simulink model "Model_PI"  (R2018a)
settings: Solver=ode15s  StartTime=0.0  StopTime=tsim  MaxStep=0.1  RelTol=1e-5
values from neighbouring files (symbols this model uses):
  C = Fc*cpc/(Fh*cph)    [calcblock.m]    (also in calcblock2.m; calcblock3.m; eNTU.m = m.c*cp.c/(m.h*cp.h); Main.m = [zeros(1,2*N-1),1])
  d0 = [Fh, Tcin, Thin]    [Main.m]    (also in Main_OL.m; runTestCalcBlk.m; runTransf.m = [Fh; Tcin; U0; Ffeed0; m0; Tfeed0]; runTransfOL.m)
  d_step = [Fh, Tcin+0, Thin*1]    [Main_OL.m]    (also in runTestCalcBlk.m = [Fh, Tcin, Thin]; Main.m = [Fh, Tcin, Thin])
  d_tstep = 300    [Main.m]    (also in Main_OL.m = 3000; runTestCalcBlk.m; runTransf.m = [500; 50000; 70000; 130000; 50000; 50000]; runTransfOL.m = [500 5000 7000 13000])
  Fc0 = 5    [Main.m]    (also in Main_OL.m; runTestCalcBlk.m; runTransf.m; runTransfOL.m)
  Kc = 1/k*tau/(tauC+theta)    (= -0.124875124875)    [Main.m]    (also in runTransf.m = 1/kM(i)*tau(i)/(tauCM(i)+theta(i)); runTransfOL.m = 1/kM(i)*tau(i)/(tauCM(i)+theta(i)))
  nd = size(d0,2)    [Main.m]    (also in Main_OL.m; runTestCalcBlk.m; runTransf.m = size(d0,1); runTransfOL.m)
  np = size(p,2)    [Main.m]    (also in Main_OL.m; runTestCalcBlk.m; runH2Psim.m = length(param); runTransf.m)
  nu = 1    [Main.m]    (also in Main_OL.m; runTestCalcBlk.m; runH2Psim.m = length(u0); runTransf.m)
  nx = size(x0,1)    [Main.m]    (also in Main_OL.m; runTestCalcBlk.m; H2P_Turbine_driven.m = param(end); runTD.m = length(x0))
  p = [N, Fc0, rhoc, rhoh,U,A,cpc,cph]    [Main.m]    (also in Main_OL.m; runTestCalcBlk.m; NonlinearMap.m = [U;A;Fc(i);Fh;cpc;cph;Tcin;Thin]; runTransf.m = [N, Fc0, rhoc, rhoh, U0, A,cpc,cph])
  tauI = min(tau,4*(tauC+theta))    [Main.m]    (also in runTransf.m = min(tau(i), 4*(tauCM(i)+theta(i))); runTransfOL.m = min(tau(i), 4*(tauCM(i)+theta(i))))
  Thsp = Thsp0+dThsp    [Main.m]    (also in Main_OL.m = sp(j); runTestCalcBlk.m; runTransf.m = Thsp0; runTransfOL.m = Thsp0)
  Thsp0 = Thend(end)    [Main.m]    (also in Main_OL.m; runTestCalcBlk.m; runTransf.m = x0(end-1);  2.971202611676064e+02; runTransfOL.m = x0(end);  2.971202611676064e+02)
  tstep = 100    [Main.m]    (also in Main_OL.m = 500; runTransf.m = 10000; runTransfOL.m)
  x0 = [Tcend(1:N)'; Thend(1:N)']    [Main.m]    (also in Main_OL.m; runTestCalcBlk.m; runTD.m = [TE0;TD0;TSh0;MD0; MSh0;w0;TA0;0;0;0;0;0;0;0;0;0]; runBD.m = [TE0;TD0;TSh0;MD0; MSh0;w0;TA0;0;0;0;0;0;0;0;0;0])
undefined symbols (not defined in the file or in its folder): HEXode

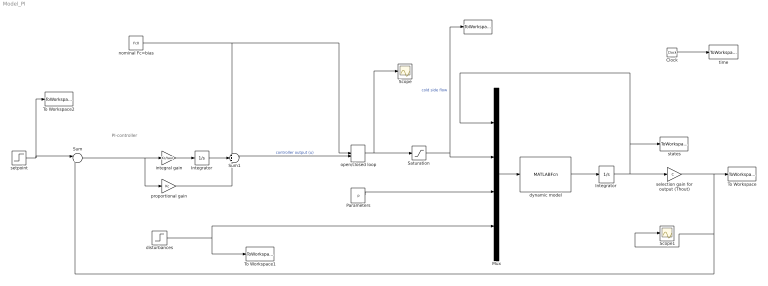
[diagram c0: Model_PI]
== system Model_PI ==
  note: PI-controller
  " " : ToWorkspace  VariableName=uc  SampleTime=-1
  Clock : Clock
  Integrator : Integrator
  "Integrator " : Integrator  InitialCondition=x0
  Mux : Mux
  Parameters : Constant  Value=p
  "Saturation " : Saturate  UpperLimit=inf  LowerLimit=0
  Scope : Scope
  Scope1 : Scope
  Sum : Sum  Inputs=|+-
  Sum1 : Sum  Inputs=+++
  To Workspace : ToWorkspace  VariableName=Thout  SampleTime=-1
  To Workspace1 : ToWorkspace  VariableName=dsim  SampleTime=-1
  To Workspace2 : ToWorkspace  VariableName=Tsp  SampleTime=-1
  disturbances : Step  Time=d_tstep  Before=d0  After=d_step  SampleTime=0
  dynamic model : MATLABFcn  MATLABFcn=HEXode(u(1:nx),u(nx+1:nx+nu),u(nx+nu+1:nx+nu+np),u(nx+nu+np+1:nx+nu+np+nd))  OutputDimensions=nx  Output1D=off
  integral gain : Gain  Gain=Kc/tauI  Multiplication=Matrix(K*u)
  nominal Fc=bias : Constant  Value=Fc0
  open/closed loop : ManualSwitch  CurrentSetting=0
  proportional gain : Gain  Gain=Kc  Multiplication=Matrix(K*u)
  selection gain for output (Thout) : Gain  Gain=C  Multiplication=Matrix(K*u)
  setpoint : Step  Time=tstep  Before=Thsp0  After=Thsp  SampleTime=0
  states : ToWorkspace  VariableName=T  SampleTime=-1
  time : ToWorkspace  VariableName=t  SampleTime=-1
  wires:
  dynamic model/1 -> "Integrator "/1
  "Integrator "/1 -> selection gain for output (Thout)/1, states/1, Mux/1
  Mux/1 -> dynamic model/1
  Clock/1 -> time/1
  Parameters/1 -> Mux/3
  disturbances/1 -> To Workspace1/1, Mux/4
  "Saturation "/1 -> Mux/2, " "/1  "cold side flow"
  Sum/1 -> proportional gain/1, integral gain/1
  integral gain/1 -> Integrator/1
  Integrator/1 -> Sum1/2
  selection gain for output (Thout)/1 -> Scope1/1, Sum/2, To Workspace/1
  open/closed loop/1 -> Scope/1, "Saturation "/1
  nominal Fc=bias/1 -> open/closed loop/1, Sum1/1
  proportional gain/1 -> Sum1/3
  Sum1/1 -> open/closed loop/2  "controller output (u)"
  setpoint/1 -> To Workspace2/1, Sum/1
